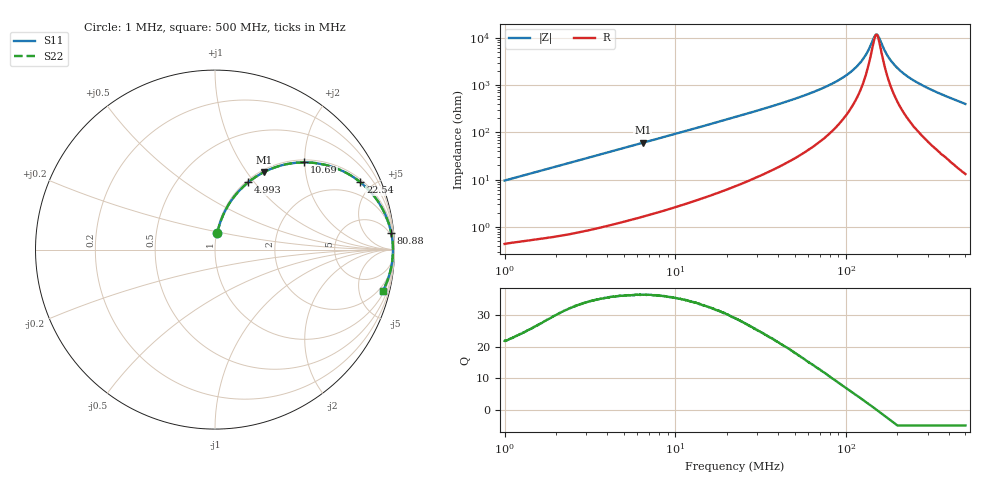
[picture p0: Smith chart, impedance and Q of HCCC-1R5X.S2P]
!s-Parameter Generated by FASTRON Sdn. Bhd.
!FASTRON P/N : HCCC-1R5X
!Keysight Technologies,E4991B,MY54100416,A.01.15
!Date: Thu Apr 02 13:43:53 2026
!Version  : Rev00 Thu Apr 02 13:43:53 2026
!Data & Calibration Information:
!PortZ  Port1:50+j0  Port2:50+j0
!When reading, reference impedance value at option line is always used.
! Remarks : This data is being provided solely for informational purposes.
!Freq	S11	S21	S12	S22
# Hz S dB R 50
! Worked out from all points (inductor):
!   1601 points, 1 MHz to 500 MHz, reference 50 ohm
!   read as one part in series: L = 1.52 uH near 1.032 MHz
!   highest Q = 36.6 at 6.452 MHz (marker M1), where L = 1.49 uH
!   self-resonance near 150.7 MHz
!   S11 on the Smith chart (normalised r, x): 1 MHz: 1.01, +0.19; 4.993 MHz: 1.03, +0.94; 10.69 MHz: 1.06, +1.99; 22.54 MHz: 1.15, +4.24; 80.88 MHz: 3, +20; 500 MHz: 1.26, -7.99
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1000000  -20.43 81.9  -0.08 -5.5  -0.08 -5.5  -20.43 81.9
2820919  -11.85 73.5  -0.36 -14.8  -0.36 -14.8  -11.85 73.5
4992965  -7.54 63.6  -0.95 -24.8  -0.95 -24.8  -7.54 63.6
6451950  -5.84 57.7  -1.45 -30.7  -1.45 -30.7  -5.84 57.7
7957584  -4.60 52.4  -2.02 -36.1  -2.02 -36.1  -4.60 52.4
1.069011e7  -3.15 44.3  -3.12 -44.1  -3.12 -44.1  -3.15 44.3
2.236068e7  -1.00 25.1  -7.46 -63.0  -7.46 -63.0  -1.00 25.1
2.253506e7  -0.99 24.9  -7.51 -63.1  -7.51 -63.1  -0.99 24.9
3.591546e7  -0.44 15.8  -11.28 -71.7  -11.28 -71.7  -0.44 15.8
6.307767e7  -0.17 8.1  -17.00 -77.9  -17.00 -77.9  -0.17 8.1
8.087875e7  -0.12 5.5  -20.34 -79.0  -20.34 -79.0  -0.12 5.5
1.005306e8  -0.09 3.5  -24.28 -78.2  -24.28 -78.2  -0.09 3.5
1.174283e8  -0.08 2.1  -28.46 -74.6  -28.46 -74.6  -0.08 2.1
1.299065e8  -0.08 1.2  -32.61 -67.3  -32.61 -67.3  -0.08 1.2
1.453951e8  -0.07 0.3  -40.00 -31.3  -40.00 -31.3  -0.07 0.3
1.494024e8  -0.07 0.1  -41.39 -7.9  -41.39 -7.9  -0.07 0.1
1.553196e8  -0.07 -0.3  -40.38 27.7  -40.38 27.7  -0.07 -0.3
1.77937e8  -0.08 -1.4  -31.69 69.8  -31.69 69.8  -0.08 -1.4
2.062371e8  -0.08 -2.7  -26.36 77.2  -26.36 77.2  -0.08 -2.7
2.523965e8  -0.10 -4.6  -21.80 79.4  -21.80 79.4  -0.10 -4.6
3.403856e8  -0.16 -8.0  -17.12 78.5  -17.12 78.5  -0.16 -8.0
5e8  -0.33 -13.9  -12.37 74.2  -12.37 74.2  -0.33 -13.9
